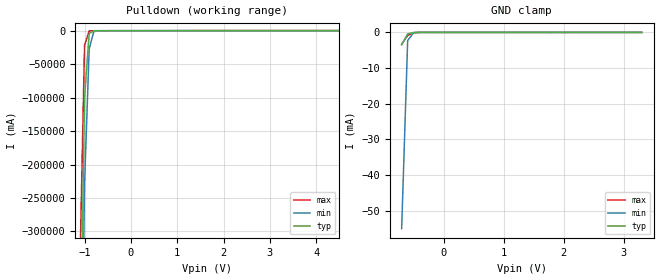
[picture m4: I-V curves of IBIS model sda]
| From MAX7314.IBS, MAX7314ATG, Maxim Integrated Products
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|   Model sda
[Model]   sda
Model_type   I/O_open_drain
|Signal   SDA
Vinh = 2.3  |0.7XV+,typ
Vinl = 1.0  |0.3XV+,typ
|   typ   min   max
C_comp   2pF   1.6pF   2.5pF
[Temperature Range]   25.00   85.00   -40
[Voltage Range]   3.30V   2V   3.6V
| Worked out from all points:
|   slope of the pulldown table from 0 to 0.495 V, typ, clamps not added: 20 ohm
|   GND clamp passes 1 mA (typ) near -0.62 V on its own axis
[GND Clamp]
|Volts   I(typ)   I(min)   I(max)
|-3.30  -2.534e+04  -2.570e+04  -2.506e+04
|-3.20  -2.383e+04  -2.420e+04  -2.354e+04
|-3.10  -2.233e+04  -2.270e+04  -2.203e+04
|-3.00  -2.083e+04  -2.121e+04  -2.052e+04
|-2.90  -1.934e+04  -1.973e+04  -1.902e+04
|-2.80  -1.786e+04  -1.826e+04  -1.752e+04
|-2.70  -1.639e+04  -1.680e+04  -1.604e+04
|-2.60  -1.494e+04  -1.535e+04  -1.457e+04
|-2.50  -1.350e+04  -1.393e+04  -1.313e+04
|-2.40  -1.211e+04  -1.254e+04  -1.173e+04
|-2.30  -1.078e+04  -1.120e+04  -1.041e+04
|-2.20  -9.577e+03  -9.944e+03  -9.282e+03
|-2.10  -8.551e+03  -8.825e+03  -8.362e+03
|-2.00  -7.668e+03  -7.865e+03  -7.516e+03
|-1.90  -6.829e+03  -7.001e+03  -6.681e+03
|-1.80  -6.002e+03  -6.171e+03  -5.849e+03
|-1.70  -5.179e+03  -5.352e+03  -5.020e+03
|-1.60  -4.362e+03  -4.541e+03  -4.196e+03
|-1.50  -3.553e+03  -3.737e+03  -3.379e+03
|-1.40  -2.754e+03  -2.946e+03  -2.571e+03
|-1.30  -1.973e+03  -2.172e+03  -1.780e+03
|-1.20  -1.224e+03  -1.429e+03  -1.021e+03
|-1.10  -5.495e+02  -7.491e+02  -3.530e+02
|-1.00  -1.006e+02  -2.297e+02  -2.160e+01
|-0.90  -4.351e+00  -2.720e+01  -2.026e-01
|-0.80  -9.694e-02  -1.368e+00  -8.380e-03
-700mV    -3.517mA   -55.04mA   -3.247mA
-600mV    -416.8uA   -2.283mA   -874.1uA
-500mV    -35.13uA   -99.79uA   -76.68uA
3.3V      0A         0A         0A
[PULLDOWN]
|Volts   I(typ)   I(min)   I(max)
-3.3V     -25.34kA   -25.7kA    -25.06kA
-1.1V     -549.5A    -749.2A    -353.1A
-1V       -100.7A    -229.7A    -21.68A
-900mV    -4.395A    -27.22A    -278.6mA
-800mV    -137.7mA   -1.391A    -78.8mA
-700mV    -40.22mA   -76.05mA   -67.14mA
6.6V      92.48mA    21.73mA    176.8mA
[Ramp]
|Variable   typ   min   max
dV/dt_r  1.96/19.80n  1.19/28.20n  2.17/15.20n
dV/dt_f  1.98/38.00n  1.19/126.00n  2.18/18.00n
R_load=4.7k
